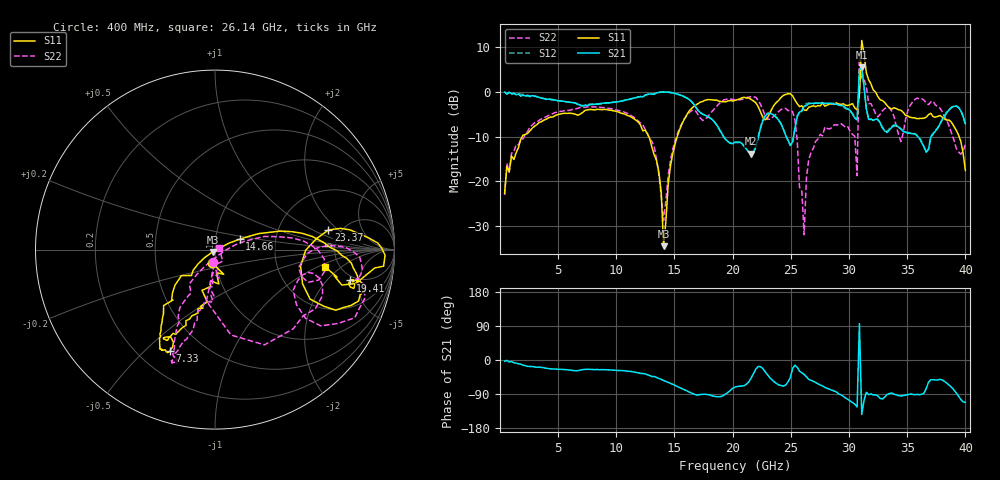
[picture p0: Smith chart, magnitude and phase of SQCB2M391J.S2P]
! Network Analyzer HP8722ES.07.66: Jul 25, 2000 Serial No. US39175408
! 27 Oct 2004  14:31:25
! Frequency  S11  S21  S12  S22
# HZ  S  DB R  50
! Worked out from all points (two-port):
!   201 points, 400 MHz to 40 GHz, reference 50 ohm
!   highest |S21| = 5.42 dB at 31.09 GHz (marker M1); lowest = -13.8 dB at 21.59 GHz (marker M2)
!   |S21| within 3 dB of the highest: 30.85 GHz to 31.23 GHz (379.8 MHz wide, 1.22 % of centre)
!   lowest |S11| = -34.4 dB at 14.06 GHz (marker M3), VSWR 1.04, Z = 48.6 - j1.29 ohm
!   |S11| at or under -10 dB: start of sweep to 1.922 GHz; 12.78 GHz to 15.24 GHz (2.455 GHz wide, 17.5 % of centre); 39.46 GHz to end of sweep
!   |S22| runs from -31.9 to 8.5 dB; largest |S21 - S12| = 0.67
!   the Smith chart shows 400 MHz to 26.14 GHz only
!   S11 on the Smith chart (normalised r, x): 400 MHz: 0.96, -0.14; 7.33 GHz: 0.33, -0.60; 14.66 GHz: 1.31, +0.15; 19.41 GHz: 4.44, -3.76; 23.37 GHz: 3.99, +1.48; 26.14 GHz: 3.89, -1.24
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4e8  -22.60 -103.2  -0.13 -3.3  -0.08 -2.8  -23.02 -99.6
7.132e9  -4.60 -113.6  -3.14 -25.4  -3.20 -26.4  -3.56 -109.2
7.33e9  -4.17 -113.9  -3.07 -24.6  -3.06 -26.1  -3.49 -110.1
1.3666e10  -18.11 -139.7  -0.18 -48.6  -0.15 -49.1  -18.63 -122.4
1.4062e10  -34.40 -135.8  -0.08 -53.6  -0.13 -54.1  -28.74 -59.5
1.4656e10  -16.58 22.8  -0.24 -61.6  -0.16 -62.5  -15.26 15.5
1.9408e10  -2.26 -12.9  -10.66 -89.5  -10.71 -89.3  -1.74 -5.2
2.02e10  -1.97 -12.4  -11.28 -71.4  -11.34 -71.8  -1.86 -11.2
2.1586e10  -1.74 -22.4  -13.82 -47.7  -13.76 -46.8  -1.13 -18.1
2.3368e10  -3.86 9.8  -4.99 -52.2  -4.95 -52.9  -5.90 -16.2
2.5348e10  -1.87 -13.6  -8.27 -13.8  -8.05 -16.3  -6.30 -79.4
2.614e10  -4.11 -9.0  -3.27 -38.1  -3.13 -38.2  -31.86 24.7
2.6932e10  -3.18 2.0  -2.61 -56.5  -2.77 -57.6  -12.62 40.6
3.0694e10  -4.06 -12.3  -6.29 -124.0  -6.22 -123.3  -18.73 -57.4
3.0892e10  -0.79 -29.3  4.83 96.0  0.81 88.0  8.50 3.8
3.109e10  11.37 -46.3  5.42 -143.7  5.09 -143.9  3.03 169.3
3.1288e10  8.51 -51.5  1.15 -106.4  1.08 -107.0  2.79 -125.8
3.1486e10  4.18 -47.5  -3.77 -85.2  -3.76 -87.1  1.18 -102.1
3.3466e10  -3.63 -109.2  -8.53 -88.6  -8.25 -89.0  -3.56 177.3
3.505e10  -5.44 -163.6  -9.27 -91.4  -9.09 -92.1  -4.31 -158.8
3.703e10  -4.83 112.4  -10.14 -52.2  -9.99 -53.4  -2.31 127.5
4e10  -17.55 64.7  -7.15 -111.8  -7.18 -112.7  -11.70 -29.1
